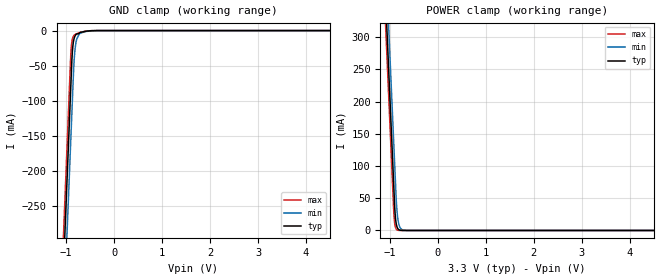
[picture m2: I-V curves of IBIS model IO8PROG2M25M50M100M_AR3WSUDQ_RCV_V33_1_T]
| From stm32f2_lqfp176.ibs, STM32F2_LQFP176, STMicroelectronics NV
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| *** New cell (Generated with 5.14beta1 (Sep 20 2010 13:23:23))
[Model]   IO8PROG2M25M50M100M_AR3WSUDQ_RCV_V33_1_T
Model_type Input
Polarity   Non-Inverting
Enable   Active-Low
| CAP_THRESHOLD on pad IOV33 is "CMOS" :
| Rising=10.0% of vddio   Falling=90.0% of vddio
| C_comp min and max val. don't necessarily correlate with the min and max pvt
| but are the smallest and greatest pad capacitance found.
| var   typ   min   max
C_comp   2.53655pF  2.40975pF  2.66965pF
Vinl = 800.0mV | Dummy value overriden by next lines
Vinh = 2.00V | Dummy value overriden by next lines
[Model Spec]
| TIME_THRESHOLD on pin ZIV33 is "CORE" :
| Rising=40.0% of vddio   Falling=60.0% of vddio
Vinl 1.48450V 1.23350V 1.61250V
Vinh 1.48450V 1.23350V 1.61250V
| variable   typ   min   max
[Temperature Range] 25.0 125.0 -40.0
| variable   typ   min   max
[Voltage Range] 3.3V 2.7V 3.6V
| variable   typ   min   max
[POWER Clamp Reference] 3.3V 2.7V 3.6V
| variable   typ   min   max
[GND Clamp Reference] 0V 0V 0V
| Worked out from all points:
|   GND clamp passes 1 mA (typ) near -0.59 V on its own axis
|   POWER clamp passes 1 mA (typ) near -0.81 V on its own axis
[POWER Clamp]
-3.3V     4.117A     4.183A     4.076A
-1.09V    360mA      425.6mA    319.3mA
-1.05V    292mA      357.6mA    251.3mA
-1.01V    224mA      289.6mA    183.3mA
-910mV    53.96mA    119.6mA    18.43mA
-900mV    36.96mA    102.6mA    11.2mA
-880mV    16.97mA    68.61mA    4.141mA
-860mV    7.791mA    38.56mA    1.53mA
-840mV    3.577mA    21.53mA    565.5uA
-780mV    346.2uA    3.745mA    28.55uA
-660mV    3.242uA    113.2uA    73.21nA
6.6V      0A         0A         0A
[GND Clamp]
-3.3V     -4.156A    -4.231A    -4.108A
-1.06V    -347.5mA   -423.2mA   -300.1mA
-940mV    -143.5mA   -219.2mA   -96.09mA
-900mV    -75.54mA   -151.2mA   -30.39mA
-880mV    -41.78mA   -117.2mA   -15.62mA
-870mV    -30.28mA   -100.2mA   -12.04mA
-840mV    -13.1mA    -50.87mA   -7.186mA
-810mV    -7.18mA    -24.07mA   -5.432mA
-780mV    -4.86mA    -12.37mA   -4.416mA
-700mV    -2.552mA   -3.603mA   -2.454mA
-350mV    -11.93uA   -60.06uA   -2.46uA
6.6V      10.25nA    1.32uA     122.8pA
